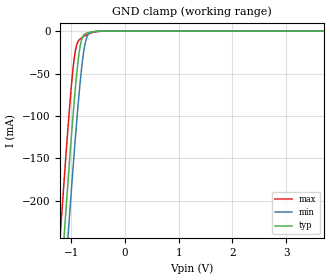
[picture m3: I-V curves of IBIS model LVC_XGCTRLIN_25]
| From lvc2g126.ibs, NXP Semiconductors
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|   Model LVC_XGCTRLIN_25
[Model]   LVC_XGCTRLIN_25
Model_type   Input
Vinl =   0.7V
Vinh =   1.7V
C_comp   2.9744pF   2.2245pF   3.8599pF
|Ambient temperature:   25   85   -40
[Temperature Range]   30   90   -35
[Voltage Range]   2.5V   2.3V   2.7V
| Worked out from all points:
|   GND clamp passes 1 mA (typ) near -0.61 V on its own axis
|Process Range   nominal   slow   fast
[GND_clamp]
| voltage   I(typ)   I(min)   I(max)
-5.5V     -4.533A    -4.59A     -4.476A
-1.208V   -311.2mA   -376.9mA   -244.9mA
-1.186V   -290.9mA   -356.6mA   -224.8mA
-1.12V    -231.1mA   -296.4mA   -165.6mA
-1.054V   -172.9mA   -237.4mA   -109.1mA
-944mV    -82.87mA   -143.4mA   -32.14mA
-900mV    -51.94mA   -108.3mA   -16.56mA
-856mV    -27.03mA   -75.74mA   -10.72mA
-768mV    -4.801mA   -24.46mA   -6.387mA
-702mV    -2.124mA   -6.152mA   -4.132mA
-400mV    -82.3uA    -86.02uA   -67.85uA
5.5V      0A         0A         0A
